| IBIS file 256bga.ibs generated by Viper version: 2014.09.14
[IBIS Ver]   4.2
[Comment Char]   |_char
[File Name]   256bga.ibs
[File Rev]   1
[Date]   Fri Apr  3 14:52:16 2015
[Source]   FSL Viper 2014.09.14
[Notes]
   Single RLC values cover parasitic for all power pins
   (of a particular power domain) combined and hence
   if there are more than one power pin, RLC values are mentioned
   only for one pin and other power pins are commented
[Disclaimer] IMPORTANT NOTICE
  This information is provided on an AS IS basis and without warranty.
  IN NO EVENT SHALL Freescale BE LIABLE FOR INCIDENTAL OR CONSEQUENTIAL
  DAMAGES ARISING FROM USE OF THIS INFORMATION. THIS DISCLAIMER OF
  WARRANTY EXTENDS TO THE USER OF THE INFORMATION, AND TO THEIR CUSTOMERS
  OR USERS OF PRODUCTS  AND IS IN LIEU OF ALL WARRANTIES WHETHER EXPRESS,
  IMPLIED, OR STATUTORY, INCLUDING IMPLIED WARRANTIES OF MERCHANTABILITY
  OR FITNESS FOR PARTICULAR PURPOSE.
  Freescale does not represent or warrant that the information furnished
  hereunder is free of infringement of any third party patents,
  copyrights, trade secrets, or other intellectual property rights.
  Freescale does not represent or warrant that the information is free of
  defect, or that it meets any particular standard, requirements or need
  of the user of the infomation or their customers.
  Freescale reserves the right to change the information in this file
  without notice.
   http://www.freescale.com
[Copyright]   (C) Copyright Freescale 2004 - 2015, All Rights Reserved.
|   BGA256
[Component]   BGA256
[Manufacturer]   FREESCALE
[Package]
| variable   typ   min   max
R_pkg   0.1964927   0.0083184   0.423379
L_pkg   3.36922nH   0.16729nH   6.71183nH
C_pkg   6.27951pF   0.85815pF   129.42pF
[Pin] signal_name   model_name   R_pin   L_pin   C_pin
A1   PC_15   pad_sr_hv   0.324213  5.52013nH 1.17247pF
A2   PB_2   pad_sr_hv   0.275249  4.67685nH 1.0835pF
A3   PC_13   pad_sr_hv   0.255357  4.27779nH 1.00875pF
A4   PI_1   pad_sr_hv   0.242099  4.05505nH 0.98353pF
A5   PE_7   pad_sr_hv   0.230813  3.88614nH 0.95807pF
A6   PH_8   pad_sr_hv   0.236383  4.04028nH 0.95422pF
A7   PE_2   pad_sr_hv   0.179001  3.25631nH 1.25499pF
A8   PE_4   pad_sr_hv   0.233047  3.75042nH 0.98335pF
A9   PC_4   pad_sr_hv   0.263865  4.60171nH 1.02217pF
A10   PE_3   pad_sr_hv   0.27758   4.42732nH 1.11798pF
A11   PH_9   pad_sr_hv   0.309578  5.31158nH 1.18041pF
A12   PI_4   pad_sr_hv   0.279418  4.43534nH 1.10534pF
A13   PH_11   pad_sr_hv   0.281574  4.54521nH 1.12217pF
A14   PE_14   pad_sr_hv   0.300351  4.79127nH 1.11754pF
A15   PA_10   pad_sr_hv   0.272795  4.57773nH 1.17751pF
A16   PG_11   pad_sr_hv   0.343998  5.8046nH  1.52808pF
B1   PH_13   pad_sr_hv   0.309012  4.60385nH 1.40593pF
B2   PC_14   pad_sr_hv   0.27654   4.18497nH 1.38321pF
B3   PC_8   pad_sr_hv   0.274109  4.57938nH 1.27321pF
B4   PC_12   pad_sr_hv   0.202262  3.43434nH 0.98387pF
B5   PI_3   pad_sr_hv   0.190194  3.28388nH 0.99610pF
B6   PE_6   pad_sr_hv   0.18691   3.23119nH 0.98134pF
B7   PH_5   pad_sr_hv   0.200167  3.3174nH  0.98670pF
B8   PE_5   pad_sr_hv   0.266098  4.16068nH 1.1138pF
B9   PC_5   pad_sr_hv   0.252578  4.0635nH  1.22285pF
B10   PC_0   pad_sr_hv   0.31327   4.95432nH 1.3505pF
B11   PC_2   pad_sr_hv   0.214991  3.6177nH  1.13299pF
B12   PH_12   pad_sr_hv   0.233157  3.75179nH 1.14785pF
B13   PG_10   pad_sr_hv   0.237631  4.02177nH 1.10873pF
B14   PA_11   pad_sr_hv   0.23566   4.05457nH 1.17578pF
B15   PA_9   pad_sr_hv   0.250805  4.21236nH 1.13432pF
B16   PA_8   pad_sr_hv   0.293828  5.20672nH 1.11636pF
C1   PH_14   pad_sr_hv   0.297223  4.25757nH 1.33977pF
C2   VDD_HV_A   POWER   0.0083184 0.16729nH 129.42pF
C3   PC_9   pad_sr_hv   0.182711  3.35963nH 1.20027pF
C4   PL_0   pad_sr_hv   0.367841  5.35885nH 1.64142pF
C5   PI_0   pad_sr_hv   0.159272  2.80972nH 1.01543pF
C6   PH_7   pad_sr_hv   0.143217  2.44485nH 0.95198pF
C7   PH_6   pad_sr_hv   0.151913  2.51215nH 0.99717pF
C8   PORST   NC   0.216992  3.34396nH 1.09417pF
|C9   VDD_HV_A   POWER
C10   PA_5   pad_sr_hv   0.152018  2.77919nH 1.12939pF
C11   PC_3   pad_sr_hv   0.161702  2.99625nH 1.19732pF
C12   PE_15   pad_sr_hv   0.17795   3.08825nH 1.10818pF
C13   PG_14   pad_sr_hv   0.253163  3.84261nH 1.24769pF
C14   PE_12   pad_sr_hv   0.201768  3.44496nH 1.16937pF
C15   PA_7   pad_sr_hv   0.23726   3.9272nH  1.07868pF
C16   PE_13   pad_sr_hv   0.279324  4.51364nH 1.11731pF
D1   PG_5   pad_sr_hv   0.268975  4.29308nH 1.11627pF
D2   PI_6   pad_sr_hv   0.246617  3.93408nH 1.15737pF
D3   PJ_4   pad_sr_hv   0.199472  3.12124nH 1.28002pF
D4   PB_3   pad_sr_hv   0.126953  2.30946nH 1.23447pF
D5   PK_15   pad_sr_hv   0.329374  5.02948nH 1.74265pF
D6   PI_2   pad_sr_hv   0.132388  2.52105nH 1.02497pF
D7   PH_4   pad_sr_hv   0.115282  1.99435nH 1.03528pF
D8   VDD_LV   POWER   0.010575  0.19674nH 30.7472pF
D9   PC_1   pad_sr_hv   0.126989  2.35316nH 1.0334pF
D10   PH_10   pad_sr_hv   0.22571   3.84732nH 1.30005pF
D11   PA_6   pad_sr_hv   0.296653  4.83515nH 1.36284pF
D12   PI_5   pad_sr_hv   0.224317  3.57931nH 1.24766pF
D13   PG_15   pad_sr_hv   0.205499  3.25677nH 1.21668pF
D14   PF_14   pad_sr_hv   0.180972  3.12583nH 1.11984pF
D15   PF_15   pad_sr_hv   0.227901  3.62451nH 1.08322pF
D16   PH_2   pad_sr_hv   0.276852  5.02354nH 1.08104pF
E1   PG_3   pad_sr_hv   0.253683  4.12842nH 1.05526pF
E2   PI_7   pad_sr_hv   0.212802  3.21299nH 1.28853pF
E3   PH_15   pad_sr_hv   0.156903  2.88238nH 1.20949pF
E4   PG_2   pad_sr_hv   0.210986  3.62346nH 1.22526pF
|E5   VDD_LV   POWER
E6   VSS   GND   NA   NA   NA
E7   PK_10   pad_sr_hv   0.231455  3.57336nH 1.58203pF
E8   PK_9   pad_sr_hv   0.210359  3.34085nH 1.55851pF
E9   PQ_5   pad_sr_hv   0.289312  5.02756nH 1.94156pF
E10   PQ_7   pad_sr_hv   0.130619  2.66962nH 1.3489pF
E11   PP_14   pad_sr_hv   0.359522  5.89452nH 1.58314pF
E12   PP_12   pad_sr_hv   0.197837  3.39949nH 1.36199pF
E13   PG_0   pad_sr_hv   0.218999  3.85566nH 1.36794pF
E14   PG_1   pad_sr_hv   0.183635  3.3765nH  1.12353pF
E15   PH_0   pad_sr_hv   0.226968  3.63885nH 1.10004pF
|E16  VDD_HV_A   POWER
F1   PA_2   pad_sr_hv   0.253018  3.97314nH 1.07913pF
F2   PG_4   pad_sr_hv   0.189338  2.99254nH 1.22241pF
F3   PA_1   pad_sr_hv   0.16757   3.006nH   1.13338pF
F4   PE_1   pad_sr_hv   0.0967521 2.00002nH 1.18987pF
F5   PQ_3   pad_sr_hv   0.173294  3.35889nH 1.13893pF
F6   PQ_4   pad_sr_hv   0.0866596 1.50689nH 1.28544pF
F7   PL_1   pad_sr_hv   0.23813   3.75952nH 1.73391pF
F8   PK_11   pad_sr_hv   0.201554  2.91847nH 1.82536pF
F9   PM_5   pad_sr_hv   0.13711   2.1568nH  1.5445pF
F10   PQ_6   pad_sr_hv   0.269385  3.86626nH 1.8232pF
F11   PP_15   pad_sr_hv   0.260423  4.77442nH 1.53805pF
F12   PP_13   pad_sr_hv   0.234499  3.79265nH 1.50588pF
F13   PH_1   pad_sr_hv   0.168736  3.12009nH 1.33014pF
F14   PH_3   pad_sr_hv   0.166241  2.94445nH 1.06608pF
F15   PG_12   pad_sr_hv   0.190384  3.12816nH 1.01871pF
F16   PG_13   pad_sr_hv   0.22642   3.59165nH 0.99739pF
G1   PE_8   pad_sr_hv   0.225749  3.72981nH 0.97317pF
G2   PE_0   pad_sr_hv   0.195397  3.11095nH 1.02224pF
G3   PE_10   pad_sr_hv   0.229783  3.89474nH 1.11855pF
G4   PA_0   pad_sr_hv   0.114046  2.41824nH 1.18032pF
G5   PQ_2   pad_sr_hv   0.216675  3.83566nH 1.46397pF
G6   VSS   GND   NA   NA   NA
G7   VSS   GND   NA   NA   NA
G8   VSS   GND   NA   NA   NA
G9   VSS   GND   NA   NA   NA
G10   VSS   GND   NA   NA   NA
G11   VSS   GND   NA   NA   NA
G12   PK_12   pad_sr_hv   0.183869  3.27482nH 1.68348pF
G13   VDD_HV_B   POWER   0.0214124 0.49257nH 2.76976pF
G14   PI_13   pad_sr_hv   0.149616  2.48634nH 0.95951pF
G15   PI_12   pad_sr_hv   0.187041  2.93315nH 1.02827pF
G16   PA_3   pad_sr_hv   0.234484  3.7268nH  0.95889pF
H1   PE_9   pad_sr_hv   0.236238  3.86112nH 1.0191pF
H2   VDD_HV_FLA   POWER   0.124151  2.47242nH 1.09009pF
H3   PE_11   pad_sr_hv   0.140229  2.58185nH 0.99036pF
H4   PK_1   pad_sr_hv   0.105626  2.33961nH 1.61172pF
H5   PQ_1   pad_sr_hv   0.169777  2.99961nH 1.84138pF
H6   VSS   GND   NA   NA   NA
H7   VSS   GND   NA   NA   NA
H8   VSS   GND   NA   NA   NA
H9   VSS   GND   NA   NA   NA
H10   VSS   GND   NA   NA   NA
H11   VSS   GND   NA   NA   NA
H12   PK_13   pad_sr_hv   0.306325  4.91077nH 1.73482pF
|H13  VDD_HV_A   POWER
|H14  VDD_LV   POWER
H15   VSS   GND   NA   NA   NA
H16   PI_11   pad_sr_hv   0.221367  3.33931nH 0.96053pF
J1   VPP   POWER   0.140209  2.92704nH 1.22854pF
J2   VRC_CTRL   NC   0.157438  3.00423nH 1.03021pF
|J3   VDD_LV   POWER
J4   PG_9   pad_sr_hv   0.111098  2.00458nH 1.12711pF
J5   PQ_0   pad_sr_hv   0.164882  3.10868nH 1.7361pF
J6   VSS   GND   NA   NA   NA
J7   VSS   GND   NA   NA   NA
J8   VSS   GND   NA   NA   NA
J9   VSS   GND   NA   NA   NA
J10   VSS   GND   NA   NA   NA
J11   VSS   GND   NA   NA   NA
J12   PK_14   pad_sr_hv   0.247754  4.27818nH 1.33171pF
J13   PD_15   pad_sr_hv   0.100917  2.05271nH 0.90159pF
J14   PI_8   pad_sr_hv   0.220627  3.54669nH 1.09326pF
J15   PI_9   pad_sr_hv   0.348494  4.82682nH 1.55356pF
J16   PI_10   pad_sr_hv   0.423379  5.81255nH 1.68207pF
K1   RESET   BD3MSCTFRESUDQ_5V0_65U_LIN   0.239361  3.85167nH 0.99574pF
K2   VDD_LP_DEC   POWER   0.161692  3.10249nH 1.19373pF
K3   PG_8   pad_sr_hv   0.139359  2.64706nH 0.95721pF
K4   PC_11   pad_sr_hv   0.105388  2.1833nH  0.95845pF
K5   PO_0   pad_sr_hv   0.115141  2.20474nH 1.1033pF
K6   VSS   GND   NA   NA   NA
K7   VSS   GND   NA   NA   NA
K8   VSS   GND   NA   NA   NA
K9   VSS   GND   NA   NA   NA
|K10  VDD_LV   POWER
|K11  VDD_LV   POWER
K12   PM_3   pad_sr_hv   0.172497  3.25455nH 1.41247pF
K13   PD_14   pad_sr_hv   0.172337  2.99427nH 1.14899pF
K14   PD_13   pad_sr_hv   0.111066  2.10931nH 1.01726pF
K15   PB_14   pad_sr_hv   0.196178  3.28502nH 1.02647pF
K16   PB_15   pad_sr_hv   0.227339  4.054nH   0.95127pF
L1   PC_10   pad_sr_hv   0.251569  4.17983nH 0.99046pF
L2   PG_7   pad_sr_hv   0.293097  4.71845nH 1.23759pF
L3   PB_0   pad_sr_hv   0.201897  3.58861nH 1.15282pF
L4   PK_2   pad_sr_hv   0.177602  3.40113nH 1.21395pF
L5   PO_1   pad_sr_hv   0.213694  3.25418nH 1.56173pF
L6   INT_BAL_SELECT   NC   0.314826  4.32886nH 1.79621pF
L7   VSS   GND   NA   NA   NA
L8   VSS   GND   NA   NA   NA
L9   VSS   GND   NA   NA   NA
|L10  VDD_LV   POWER
|L11  VDD_LV   POWER
L12   PM_4   pad_sr_hv   0.172068  3.14705nH 1.40233pF
L13   PD_12   pad_sr_hv   0.166101  3.4438nH  1.20226pF
L14   PB_12   pad_sr_hv   0.15503   2.59999nH 0.98002pF
L15   PB_13   pad_sr_hv   0.194606  3.33916nH 0.99569pF
L16   VDD_HV_ADC1   POWER   0.206943  3.7532nH  15.7874pF
M1   PG_6   pad_sr_hv   0.283502  4.49753nH 1.09148pF
M2   PB_1   pad_sr_hv   0.205532  3.68976nH 1.00559pF
M3   PK_4   pad_sr_hv   0.152284  2.97463nH 1.00496pF
M4   PF_9   pad_sr_hv   0.118913  2.5493nH  1.07247pF
M5   PK_5   pad_sr_hv   0.132422  2.67451nH 1.14673pF
M6   PK_6   pad_sr_hv   0.0666283 1.38902nH 1.22473pF
M7   PK_7   pad_sr_hv   0.0865669 1.85981nH 1.23011pF
M8   PK_8   pad_sr_hv   0.100542  2.15819nH 1.61714pF
M9   VIN1_CMP_REF   POWER   0.215054  3.65395nH 1.58105pF
M10   VDD_HV_C   POWER   0.117269  2.34843nH 1.18298pF
M11   VDD_HV_ADC1_REF   POWER   0.0787059 1.44124nH 1.27707pF
M12   PM_14   pad_sr_hv   0.209894  3.92408nH 1.63668pF
M13   PB_11   pad_sr_hv   0.092883  1.97409nH 1.07298pF
M14   PD_10   ISATWINJUDQ_5V0_65U_LIN   0.175432  3.15863nH 1.00195pF
M15   PD_11   ISATWINJUDQ_5V0_65U_LIN   0.220486  3.52758nH 1.00232pF
M16   VSS_HV_ADC1   GND   NA   NA   NA
N1   PK_3   pad_sr_hv   0.248039  4.34462nH 1.10855pF
N2   PF_8   pad_sr_hv   0.206957  3.71245nH 1.01574pF
N3   PC_6   pad_sr_hv   0.169368  2.72648nH 1.13397pF
N4   PC_7   pad_sr_hv   0.135748  2.28915nH 1.16513pF
N5   PJ_13   pad_sr_hv   0.150967  2.39633nH 1.42526pF
|N6   VDD_HV_A   POWER
N7   PB_10   pad_sr_hv   0.165253  2.68372nH 1.13243pF
N8   PF_6   pad_sr_hv   0.126268  2.48231nH 1.26737pF
|N9   VDD_HV_A   POWER
N10   PJ_1   pad_sr_hv   0.117738  2.26137nH 1.12471pF
N11   PD_2   ISATWINJUDQ_5V0_65U_LIN   0.188348  3.50853nH 1.12627pF
N12   PJ_5   pad_sr_hv   0.141933  2.80036nH 0.93565pF
N13   PB_5   ISATWINJUDQ_5V0_65U_LIN   0.146827  2.95495nH 1.12481pF
N14   PB_6   ISATWINJUDQ_5V0_65U_LIN   0.190888  3.5124nH  1.09221pF
N15   PJ_6   pad_sr_hv   0.281979  5.36611nH 1.4107pF
N16   PD_9   ISATWINJUDQ_5V0_65U_LIN   0.270608  4.61912nH 1.01224pF
P1   PF_12   pad_sr_hv   0.265582  4.10041nH 1.20373pF
P2   PF_10   pad_sr_hv   0.234967  3.59655nH 1.26762pF
P3   PF_13   pad_sr_hv   0.213758  3.76105nH 1.21205pF
P4   PA_14   pad_sr_hv   0.184951  3.37178nH 1.22458pF
P5   PJ_9   pad_sr_hv   0.19174   2.91808nH 1.17499pF
P6   PA_12   pad_sr_hv   0.151976  2.44212nH 1.02094pF
P7   PF_0   pad_sr_hv   0.215651  3.46354nH 1.17639pF
P8   PF_5   pad_sr_hv   0.138826  2.67081nH 1.15823pF
P9   PF_7   pad_sr_hv   0.14345   2.61868nH 1.09175pF
P10   PJ_3   pad_sr_hv   0.132324  2.45802nH 1.03754pF
P11   PI_15   pad_sr_hv   0.151317  2.71938nH 0.94272pF
P12   PD_4   ISATWINJUDQ_5V0_65U_LIN   0.125245  3.05062nH 1.01639pF
P13   PD_7   ISATWINJUDQ_5V0_65U_LIN   0.178694  3.76996nH 1.04848pF
P14   PD_8   ISATWINJUDQ_5V0_65U_LIN   0.169743  3.58185nH 1.17837pF
P15   PJ_8   pad_sr_hv   0.294035  5.47985nH 1.38242pF
P16   PJ_7   pad_sr_hv   0.371712  6.71183nH 1.44669pF
R1   PF_11   pad_sr_hv   0.298674  4.95116nH 1.14179pF
R2   PA_15   pad_sr_hv   0.276213  4.59399nH 1.20961pF
R3   PJ_11   pad_sr_hv   0.253131  4.179nH   1.17749pF
R4   PJ_15   pad_sr_hv   0.21838   3.60367nH 1.05161pF
R5   PA_13   pad_sr_hv   0.195904  3.85319nH 0.91075pF
R6   PF_2   pad_sr_hv   0.252429  4.07313nH 1.24959pF
R7   PF_3   pad_sr_hv   0.153857  3.11044nH 1.09607pF
R8   PF_4   pad_sr_hv   0.168972  3.37355nH 1.28851pF
|R9   VDD_HV_A   POWER
R10   PJ_2   pad_sr_hv   0.17194   3.0584nH  1.05184pF
R11   PJ_0   pad_sr_hv   0.193458  3.23855nH 1.01611pF
R12   PD_0   ISATWINJUDQ_5V0_65U_LIN   0.215667  4.15951nH 0.95803pF
R13   PD_3   ISATWINJUDQ_5V0_65U_LIN   0.220746  4.47397nH 1.00507pF
R14   PD_6   ISATWINJUDQ_5V0_65U_LIN   0.25805   5.35393nH 1.1348pF
R15   VDD_HV_ADC0   POWER   0.185059  3.59177nH 1.35453pF
R16   PB_7   ISATWINJUDQ_5V0_65U_LIN   0.287177  4.88948nH 1.08927pF
T1   PJ_12   pad_sr_hv   0.306594  5.1534nH  1.2548pF
T2   PA_4   pad_sr_hv   0.290128  4.77812nH 1.13216pF
T3   PK_0   pad_sr_hv   0.243555  4.00518nH 1.10005pF
T4   PJ_14   pad_sr_hv   0.25437   4.58589nH 0.986pF
T5   PJ_10   pad_sr_hv   0.207415  3.91889nH 0.93288pF
T6   PF_1   pad_sr_hv   0.283899  4.90136nH 1.21346pF
T7   XTAL   NC   0.186798  3.03261nH 0.85815pF
T8   EXTAL   NC   0.179706  2.9088nH  0.85897pF
T9   VSS   GND   NA   NA   NA
T10   PB_9   ISATWINJUDQ_5V0_65U_LIN   0.253421  3.78227nH 1.03717pF
T11   PB_8   ISATWINJUDQ_5V0_65U_LIN   0.277579  4.23821nH 1.10653pF
T12   PI_14   pad_sr_hv   0.240863  3.94095nH 0.91030pF
T13   PD_1   ISATWINJUDQ_5V0_65U_LIN   0.275986  5.53nH   1.03275pF
T14   PD_5   ISATWINJUDQ_5V0_65U_LIN   0.301236  5.97298nH 1.05914pF
T15   VSS_HV_ADC0   GND   NA   NA   NA
T16   PB_4   ISATWINJUDQ_5V0_65U_LIN   0.336521  6.16767nH 1.26785pF
[Pin Mapping]   pulldown_ref   pullup_ref
A1   VSS   VDD_HV_A
A2   VSS   VDD_HV_A
A3   VSS   VDD_HV_A
A4   VSS   VDD_HV_A
A5   VSS   VDD_HV_A
A6   VSS   VDD_HV_A
A7   VSS   VDD_HV_A
A8   VSS   VDD_HV_A
A9   VSS   VDD_HV_A
A10   VSS   VDD_HV_A
A11   VSS   VDD_HV_A
A12   VSS   VDD_HV_A
A13   VSS   VDD_HV_A
A14   VSS   VDD_HV_A
A15   VSS   VDD_HV_B
A16   VSS   VDD_HV_A
B1   VSS   VDD_HV_A
B2   VSS   VDD_HV_A
B3   VSS   VDD_HV_A
B4   VSS   VDD_HV_A
B5   VSS   VDD_HV_A
B6   VSS   VDD_HV_A
B7   VSS   VDD_HV_A
B8   VSS   VDD_HV_A
B9   VSS   VDD_HV_A
B10   VSS   VDD_HV_A
B11   VSS   VDD_HV_A
B12   VSS   VDD_HV_A
B13   VSS   VDD_HV_A
B14   VSS   VDD_HV_B
B15   VSS   VDD_HV_B
B16   VSS   VDD_HV_B
C1   VSS   VDD_HV_A
C2   NC   VDD_HV_A
C3   VSS   VDD_HV_A
C4   VSS   VDD_HV_A
C5   VSS   VDD_HV_A
C6   VSS   VDD_HV_A
C7   VSS   VDD_HV_A
C8   NC   NC
C10   VSS   VDD_HV_A
C11   VSS   VDD_HV_A
C12   VSS   VDD_HV_A
C13   VSS   VDD_HV_A
C14   VSS   VDD_HV_B
C15   VSS   VDD_HV_B
C16   VSS   VDD_HV_B
D1   VSS   VDD_HV_A
D2   VSS   VDD_HV_A
D3   VSS   VDD_HV_A
D4   VSS   VDD_HV_A
D5   VSS   VDD_HV_A
D6   VSS   VDD_HV_A
D7   VSS   VDD_HV_A
D8   NC   VDD_LV
D9   VSS   VDD_HV_A
D10   VSS   VDD_HV_A
D11   VSS   VDD_HV_A
D12   VSS   VDD_HV_A
D13   VSS   VDD_HV_A
D14   VSS   VDD_HV_B
D15   VSS   VDD_HV_B
D16   VSS   VDD_HV_B
E1   VSS   VDD_HV_A
E2   VSS   VDD_HV_A
E3   VSS   VDD_HV_A
E4   VSS   VDD_HV_A
E6   VSS   NC
E7   VSS   VDD_HV_A
E8   VSS   VDD_HV_A
E9   VSS   VDD_HV_A
E10   VSS   VDD_HV_A
E11   VSS   VDD_HV_A
E12   VSS   VDD_HV_A
E13   VSS   VDD_HV_B
E14   VSS   VDD_HV_B
E15   VSS   VDD_HV_B
F1   VSS   VDD_HV_A
F2   VSS   VDD_HV_A
F3   VSS   VDD_HV_A
F4   VSS   VDD_HV_A
F5   VSS   VDD_HV_A
F6   VSS   VDD_HV_A
F7   VSS   VDD_HV_B
F8   VSS   VDD_HV_A
F9   VSS   VDD_HV_B
F10   VSS   VDD_HV_A
F11   VSS   VDD_HV_A
F12   VSS   VDD_HV_A
F13   VSS   VDD_HV_B
F14   VSS   VDD_HV_B
F15   VSS   VDD_HV_B
F16   VSS   VDD_HV_B
G1   VSS   VDD_HV_A
G2   VSS   VDD_HV_A
G3   VSS   VDD_HV_A
G4   VSS   VDD_HV_A
G5   VSS   VDD_HV_A
G6   VSS   NC
G7   VSS   NC
G8   VSS   NC
G9   VSS   NC
G10   VSS   NC
G11   VSS   NC
G12   VSS   VDD_HV_A
G13   NC   VDD_HV_B
G14   VSS   VDD_HV_B
G15   VSS   VDD_HV_B
G16   VSS   VDD_HV_B
H1   VSS   VDD_HV_A
H2   NC   VDD_HV_FLA
H3   VSS   VDD_HV_A
H4   VSS   VDD_HV_A
H5   VSS   VDD_HV_A
H6   VSS   NC
H7   VSS   NC
H8   VSS   NC
H9   VSS   NC
H10   VSS   NC
H11   VSS   NC
H12   VSS   VDD_HV_A
H15   VSS   NC
H16   VSS   VDD_HV_B
J1   NC   VPP
J2   NC   NC
J4   VSS   VDD_HV_A
J5   VSS   VDD_HV_A
J6   VSS   NC
J7   VSS   NC
J8   VSS   NC
J9   VSS   NC
J10   VSS   NC
J11   VSS   NC
J12   VSS   VDD_HV_A
J13   VSS   VDD_HV_C
J14   VSS   VDD_HV_C
J15   VSS   VDD_HV_A
J16   VSS   VDD_HV_A
K1   VSS   VDD_HV_A
K2   NC   VDD_LP_DEC
K3   VSS   VDD_HV_A
K4   VSS   VDD_HV_A
K5   VSS   VDD_HV_A
K6   VSS   NC
K7   VSS   NC
K8   VSS   NC
K9   VSS   NC
K12   VSS   VDD_HV_B
K13   VSS   VDD_HV_C
K14   VSS   VDD_HV_A
K15   VSS   VDD_HV_C
K16   VSS   VDD_HV_C
L1   VSS   VDD_HV_A
L2   VSS   VDD_HV_A
L3   VSS   VDD_HV_A
L4   VSS   VDD_HV_A
L5   VSS   VDD_HV_A
L6   NC   NC
L7   VSS   NC
L8   VSS   NC
L9   VSS   NC
L12   VSS   VDD_HV_B
L13   VSS   VDD_HV_A
L14   VSS   VDD_HV_A
L15   VSS   VDD_HV_C
L16   NC   VDD_HV_ADC1
M1   VSS   VDD_HV_A
M2   VSS   VDD_HV_A
M3   VSS   VDD_HV_A
M4   VSS   VDD_HV_A
M5   VSS   VDD_HV_A
M6   VSS   VDD_HV_A
M7   VSS   VDD_HV_A
M8   VSS   VDD_HV_A
M9   NC   VIN1_CMP_REF
M10   NC   VDD_HV_C
M11   NC   VDD_HV_ADC1_REF
M12   VSS   VDD_HV_B
M13   VSS   VDD_HV_A
M14   VSS   VDD_HV_A
M15   VSS   VDD_HV_A
M16   VSS   NC
N1   VSS   VDD_HV_A
N2   VSS   VDD_HV_A
N3   VSS   VDD_HV_A
N4   VSS   VDD_HV_A
N5   VSS   VDD_HV_A
N7   VSS   VDD_HV_A
N8   VSS   VDD_HV_A
N10   VSS   VDD_HV_A
N11   VSS   VDD_HV_A
N12   VSS   VDD_HV_A
N13   VSS   VDD_HV_A
N14   VSS   VDD_HV_A
N15   VSS   VDD_HV_A
N16   VSS   VDD_HV_A
P1   VSS   VDD_HV_A
P2   VSS   VDD_HV_A
P3   VSS   VDD_HV_A
P4   VSS   VDD_HV_A
P5   VSS   VDD_HV_A
P6   VSS   VDD_HV_A
P7   VSS   VDD_HV_A
P8   VSS   VDD_HV_A
P9   VSS   VDD_HV_A
P10   VSS   VDD_HV_A
P11   VSS   VDD_HV_A
P12   VSS   VDD_HV_A
P13   VSS   VDD_HV_A
P14   VSS   VDD_HV_A
P15   VSS   VDD_HV_A
P16   VSS   VDD_HV_A
R1   VSS   VDD_HV_A
R2   VSS   VDD_HV_A
R3   VSS   VDD_HV_A
R4   VSS   VDD_HV_A
R5   VSS   VDD_HV_A
R6   VSS   VDD_HV_A
R7   VSS   VDD_HV_A
R8   VSS   VDD_HV_A
R10   VSS   VDD_HV_A
R11   VSS   VDD_HV_A
R12   VSS   VDD_HV_A
R13   VSS   VDD_HV_A
R14   VSS   VDD_HV_A
R15   NC   VDD_HV_ADC0
R16   VSS   VDD_HV_A
T1   VSS   VDD_HV_A
T2   VSS   VDD_HV_A
T3   VSS   VDD_HV_A
T4   VSS   VDD_HV_A
T5   VSS   VDD_HV_A
T6   VSS   VDD_HV_A
T7   NC   NC
T8   NC   NC
T9   VSS   NC
T10   VSS   VDD_HV_A
T11   VSS   VDD_HV_A
T12   VSS   VDD_HV_A
T13   VSS   VDD_HV_A
T14   VSS   VDD_HV_A
T15   VSS   NC
T16   VSS   VDD_HV_A
|*   Model Selector   *
[Model Selector] BD3MSCTFRESUDQ_5V0_65U_LIN
BD3MSCTFRESUDQ_5V0_65U_LIN_0   ipp_ttl_lv=0 CMOS Receiver
BD3MSCTFRESUDQ_5V0_65U_LIN_1   ipp_ttl_lv=1 TTL  Receiver
[Model Selector] ISATWINJUDQ_5V0_65U_LIN
ISATWINJUDQ_5V0_65U_LIN_0   ipp_ttl_lv=0 ; Automotive mode receiver
ISATWINJUDQ_5V0_65U_LIN_1   ipp_ttl_lv=1 ; TTL receiver
[Model Selector] pad_sr_hv
sr11_5v   5V VDDE, full drive
sr11_3v   3.3V VDDE, full drive
sr10_5v   5V VDDE, half drive
sr10_3v   3.3V VDDE, half drive
srin_5v   5V VDDE, input
srin_3v   3.3V VDDE, input
| End [Component] BGA256
| Models and submodels in the file (10): BD3MSCTFRESUDQ_5V0_65U_LIN_0 (I/O_open_drain), BD3MSCTFRESUDQ_5V0_65U_LIN_1 (I/O_open_drain), ISATWINJUDQ_5V0_65U_LIN_0 (Input), ISATWINJUDQ_5V0_65U_LIN_1 (Input), sr10_3v (3-state), sr10_5v (3-state), sr11_3v (3-state), sr11_5v (3-state), srin_3v (Input), srin_5v (Input)
